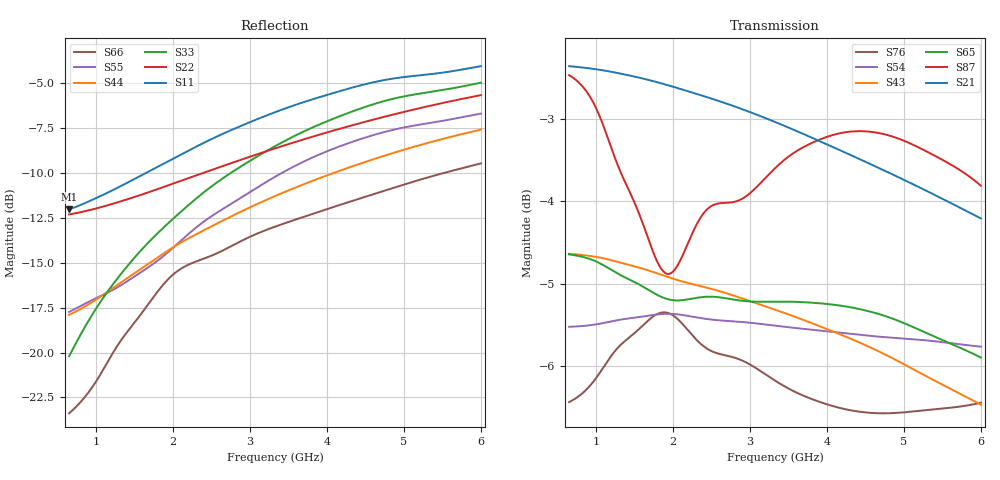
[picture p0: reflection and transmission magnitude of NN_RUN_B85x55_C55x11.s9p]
! IGNION VIRTUAL ANTENNA LIBRARY
! NN_RUN_B85x55_C55x11
! Virtual Antenna™ RUN mXTEND™: NN02-224 12.0 mm x 3.0 mm x 2.4 mm
! https://ignion.io/product/run-mxtend/
! Board: 85 mm x 55 mm
! Clearance Area: 55 mm x 11 mm
! Feeding line: L-shape; 11mm x 2mm and 5mm x 2mm
! Applications: Fleet management, IoT
! Frequency range 0.65GHz to 6GHz, step 10MHz
! Number of ports 9
! This product and its use is protected by at least one or more of the following patents and patent
! applications US 8,203,492 B2; US 8,237,615 B2; PCT/EP2013/064692; WO 2014/012842 A1; US 2019/190122 A1;
! US 62/072,671; and other domestic and international patents pending. Additional information about
! patents related to this product is available at https://ignion.io/files/Patent-list-NN.pdf, all
! rights reserved. Copyright, Ignion 2021.
! Need more help? Your platform is much different than these examples in the manual? Use our
! Fast Track service (https://ignion.io/fast-track/), for free, and get a personalized antenna design in
! just 24 hours.
! Touchstone port 1 = "Series Port"
! Touchstone port 2 = "Shunt Port"
! Touchstone port 3 = "Series Port"
! Touchstone port 4 = "Shunt Port"
! Touchstone port 5 = "Series Port"
! Touchstone port 6 = "Shunt Port"
! Touchstone port 7 = "Series Port"
! Touchstone port 8 = "Shunt Port"
! Touchstone port 9 = "Series Port"
! IE3D S-Parameters Output Version 2.0
# GHZ S MA R 50
! Nport = 9
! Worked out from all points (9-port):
!   536 points, 650 MHz to 6 GHz, reference 50 ohm
!   strongest paths, dB at 650 MHz, 1.99 GHz, 3.33 GHz, 4.67 GHz, 6 GHz:
!     S21: -2.4, -2.6, -3.0, -3.6, -4.2
!     S87: -2.5, -4.9, -3.6, -3.2, -3.8
!     S65: -4.6, -5.2, -5.2, -5.4, -5.9
!     S43: -4.6, -4.9, -5.3, -5.8, -6.5
!     S54: -5.5, -5.4, -5.5, -5.6, -5.8
!     S76: -6.4, -5.4, -6.2, -6.6, -6.4
!   lowest |S11| = -12.0 dB at 650 MHz (marker M1), VSWR 1.67, Z = 31.1 + j7.72 ohm
!   |S11| at or under -10 dB: start of sweep to 1.651 GHz
